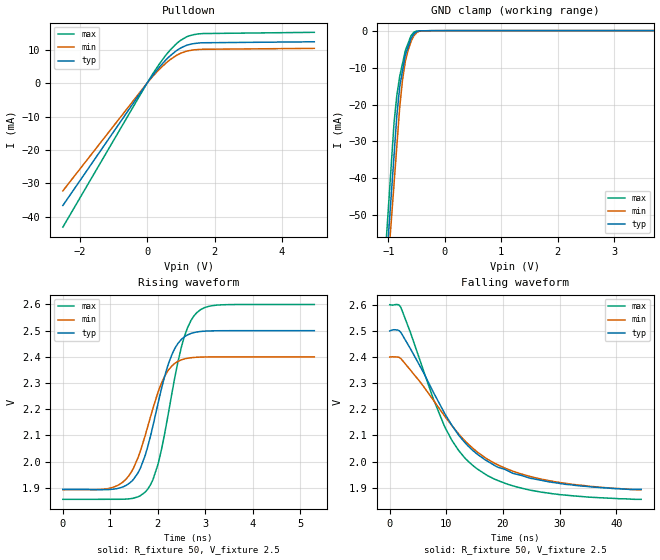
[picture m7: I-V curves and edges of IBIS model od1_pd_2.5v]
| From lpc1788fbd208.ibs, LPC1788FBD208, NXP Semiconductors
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[Model]   od1_pd_2.5v
Model_type I/O_open_drain
Vinl=7.500E-01
Vinh=1.750E+00
Vref=2.500E+00
Rref=2.000E+03
Cref=0.000E+00
Vmeas=1.250E+00
C_comp   1.240E-12   1.180E-12   1.300E-12
[Voltage Range]   2.500E+00   2.400E+00   2.600E+00
[POWER Clamp Reference]   2.500E+00   2.400E+00   2.600E+00
[GND Clamp Reference]   0.000E+00   0.000E+00   0.000E+00
[Pullup Reference]   2.500E+00   2.400E+00   2.600E+00
[Pulldown Reference]   0.000E+00   0.000E+00   0.000E+00
[Temperature Range]   25   85   -40
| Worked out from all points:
|   slope of the pulldown table from 0 to 0.375 V, typ, clamps not added: 76.6 ohm
|   GND clamp passes 1 mA (typ) near -0.55 V on its own axis
|   rising waveform, R_fixture 50, V_fixture 2.5: 20-80 % time 518ps typ, 542ps min, 493ps max; typ from 1.89 V to 2.5 V
|   falling waveform, R_fixture 50, V_fixture 2.5: 20-80 % time 11.3ns typ, 12.9ns min, 9.37ns max; typ from 2.5 V to 1.89 V
[GND Clamp]
-2.5V     -381.4mA   -371.5mA   -393.2mA
-900mV    -33.63mA   -41.3mA    -24.8mA
-850mV    -22.77mA   -30.98mA   -17.38mA
-800mV    -15.14mA   -20.67mA   -12.36mA
-750mV    -10.83mA   -13.28mA   -8.858mA
-700mV    -6.525mA   -8.291mA   -5.352mA
-650mV    -4.333mA   -5.277mA   -3.365mA
-600mV    -2.14mA    -2.967mA   -1.379mA
-550mV    -873.5uA   -1.422mA   -434.8uA
-450mV    -57.55uA   -158uA     -76.16uA
-225mV    -9.459uA   -6.37uA    -2.898uA
5V        20uA       33.33uA    12.5uA
[Pulldown]
-2.5V     -36.61mA   -32.23mA   -43.08mA
172.9mV   2.386mA    2.077mA    2.845mA
611.7mV   7.486mA    6.438mA    9.04mA
930.8mV   10.09mA    8.595mA    12.29mA
1.25V     11.52mA    9.708mA    14.13mA
1.609V    12.03mA    10.08mA    14.78mA
4.96V     12.34mA    10.38mA    15.17mA
[Rising Waveform]
R_fixture = 50
V_fixture = 2.5
V_fixture_min = 2.4
V_fixture_max = 2.6
0s        1.894V     1.893V     1.856V
1.25ns    1.902V     1.92V      1.856V
1.585ns   1.957V     2.015V     1.865V
1.783ns   2.053V     2.13V      1.893V
2.031ns   2.242V     2.277V     2.008V
2.3ns     2.409V     2.366V     2.262V
2.576ns   2.478V     2.393V     2.486V
2.7ns     2.489V     2.397V     2.539V
2.9ns     2.497V     2.399V     2.58V
5.301ns   2.5V       2.4V       2.6V
[Falling Waveform]
R_fixture = 50
V_fixture = 2.5
V_fixture_min = 2.4
V_fixture_max = 2.6
0s        2.5V       2.4V       2.6V
1.948ns   2.494V     2.394V     2.59V
7.691ns   2.266V     2.236V     2.24V
9.589ns   2.189V     2.177V     2.139V
12.04ns   2.105V     2.11V      2.047V
15.03ns   2.036V     2.044V     1.979V
18.93ns   1.98V      1.99V      1.929V
24.72ns   1.937V     1.944V     1.891V
32.45ns   1.91V      1.913V     1.869V
44.4ns    1.894V     1.893V     1.856V
[Ramp]
dV/dt_r   3.6354E-01/5.1510E-10   3.0443E-01/5.3810E-10   4.4652E-01/4.9250E-10
dV/dt_f   3.6354E-01/1.1265E-08   3.0443E-01/1.2924E-08   4.4652E-01/9.3583E-09
R_load = 50
